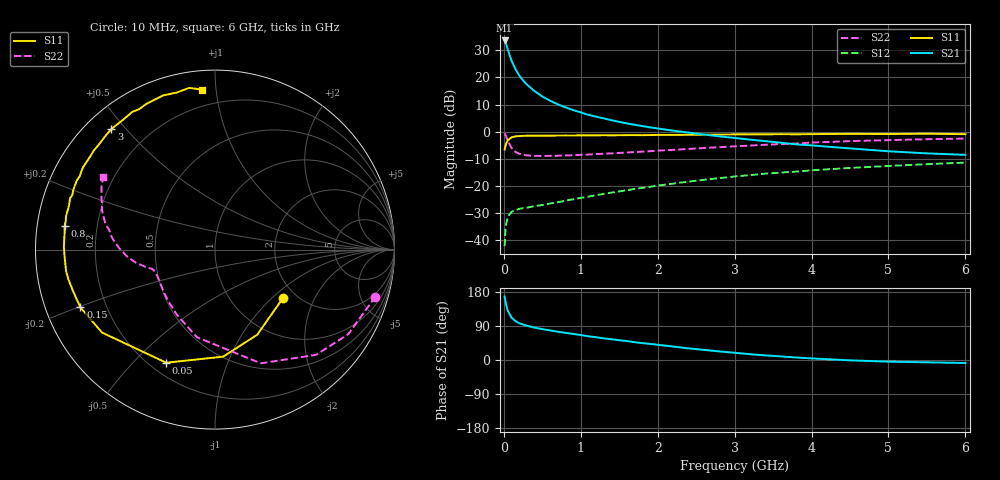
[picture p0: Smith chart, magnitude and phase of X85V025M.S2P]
! SIEMENS Small Signal Semiconductors
! BFP136W
! Si NPN RF Bipolar Junction Transistor in SOT343
! VCE = 5 V  IC = 25 mA
! Common Emitter S-Parameters:  September  1994
# GHz  S  MA  R  50
!  f  S11  S21  S12  S22
! GHz  MAG  ANG  MAG  ANG  MAG  ANG  MAG  ANG
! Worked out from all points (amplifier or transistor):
!   40 points, 10 MHz to 6 GHz, reference 50 ohm
!   highest |S21| = 33.7 dB at 10 MHz (marker M1)
!   |S21| within 3 dB of that: start of sweep to 47.28 MHz
!   unconditionally stable (mu >= 1): 856.7 MHz to 2.79 GHz
!   at 200 MHz: K = 0.37, MSG = 24.7 dB, |S12| = -28.6 dB
!   at 1.5 GHz: K = 1.13, MAG = 10.6 dB, |S12| = -22.1 dB
!   at 6 GHz: K = 0.96, MSG = 1.4 dB, |S12| = -11.5 dB
!   S11 on the Smith chart (normalised r, x): 10 MHz: 1.71, -1.18; 50 MHz: 0.26, -0.63; 150 MHz: 0.11, -0.20; 800 MHz: 0.08, +0.08; 3 GHz: 0.07, +0.46; 6 GHz: 0.10, +0.92
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0.01  0.4651 -35.4  48.37 167.4  0.0076 76.8  0.9315 -16.3
0.02  0.5293 -63.6  44.78 155.5  0.0142 66.9  0.8796 -32.4
0.03  0.5982 -85.6  41.4 145.7  0.0195 58.5  0.8132 -46.1
0.05  0.6862 -113.3  33.23 130.6  0.0262 44.8  0.6828 -68.1
0.1  0.7809 -143.7  20.44 111.8  0.0328 32.0  0.4982 -101.7
0.15  0.8162 -156.8  14.32 102.7  0.0353 28.2  0.4212 -120.1
0.2  0.824 -163.6  10.88 97.2  0.0372 26.7  0.3889 -131.7
0.25  0.8335 -168.6  8.814 93.3  0.0383 27.2  0.3728 -139.4
0.3  0.8383 -171.8  7.396 90.4  0.0391 27.6  0.3627 -144.8
0.4  0.8389 -177.2  5.583 85.4  0.0419 30.4  0.3554 -151.7
0.5  0.8419 179.1  4.456 81.4  0.0439 32.8  0.354 -156.0
0.6  0.842 176.4  3.717 78.1  0.0467 35.7  0.3552 -158.6
0.7  0.8433 173.3  3.205 74.6  0.0493 38.3  0.3576 -160.2
0.8  0.8483 171.2  2.803 71.7  0.0528 40.6  0.3612 -161.6
1.1  0.8492 164.4  2.04 62.5  0.0627 46.0  0.3767 -164.0
1.6  0.8592 155.0  1.414 49.9  0.0822 50.7  0.4101 -167.2
2.2  0.8666 144.6  1.04 35.5  0.1091 51.6  0.4588 -172.0
3  0.8861 130.6  0.763 19.0  0.1475 48.0  0.5329 179.3
3.2  0.8853 127.2  0.709 15.3  0.1567 46.6  0.5503 176.8
4.5  0.9064 108.6  0.488 -0.9  0.2125 35.8  0.6659 160.9
5.5  0.9124 99.1  0.395 -6.1  0.2495 27.6  0.7224 151.1
6  0.8946 94.7  0.371 -7.9  0.2674 23.1  0.742 147.0
